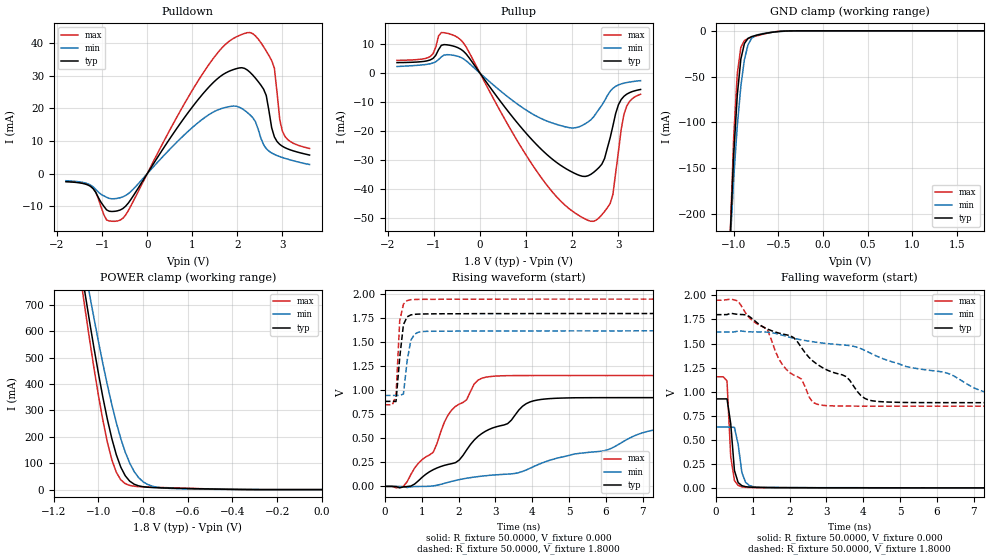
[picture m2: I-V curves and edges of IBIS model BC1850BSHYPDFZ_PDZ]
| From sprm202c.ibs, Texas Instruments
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|   Model BC1850BSHYPDFZ_PDZ
[Model]   BC1850BSHYPDFZ_PDZ
Model_type   I/O
Polarity   Non-Inverting
Enable   Active-Low
Vinl =   0.8500V
Vinh =   0.9800V
Vmeas =   0.9000V
Cref =  15.0000pF
Rref = 100.0000M
Vref =  0.000V
C_comp   1.3000pF   1.4700pF   0.9900pF
[Model Spec]
|   typ   min   max
Vinh   0.98V   0.86V   1.1V
Vinl   0.85V   0.70V   0.91V
[Temperature Range]   25.0000   0.1250k   -40.0000
[Voltage Range]   1.8000V   1.6200V   1.9500V
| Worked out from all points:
|   slope of the pulldown table from 0 to 0.27 V, typ, clamps not added: 46 ohm
|   slope of the pullup table from 0 to 0.27 V, typ, clamps not added: 44.9 ohm
|   GND clamp passes 1 mA (typ) near -0.52 V on its own axis
|   POWER clamp passes 1 mA (typ) near -0.40 V on its own axis
|   rising waveform, R_fixture 50.0000, V_fixture 0.000: 20-80 % time 2.15ns typ, 3.4ns min, 1.36ns max; typ from 0 V to 0.924 V
|   rising waveform, R_fixture 50.0000, V_fixture 1.8000: 20-80 % time 141ps typ, 150ps min, 87.9ps max; typ from 0.885 V to 1.8 V
|   falling waveform, R_fixture 50.0000, V_fixture 0.000: 20-80 % time 128ps typ, 165ps min, 115ps max; typ from 0.924 V to 0 V
|   falling waveform, R_fixture 50.0000, V_fixture 1.8000: 20-80 % time 2.09ns typ, 3.37ns min, 1.38ns max; typ from 1.8 V to 0.885 V
[Pulldown]
| voltage   I(typ)   I(min)   I(max)
-1.8V     -2.432mA   -2.13mA    -2.324mA
-1.2V     -4.535mA   -3.994mA   -4.328mA
-900mV    -11.04mA   -7.186mA   -14.12mA
-540mV    -10.64mA   -7.052mA   -13.61mA
1.32V     25.76mA    17.6mA     32.41mA
2.22V     31.69mA    18.71mA    43.1mA
2.58V     25.85mA    8.892mA    38.8mA
2.76V     14.03mA    6.343mA    34.57mA
2.82V     11.26mA    5.911mA    32.25mA
2.94V     8.959mA    5.236mA    16.41mA
3.06V     7.924mA    4.688mA    11.3mA
3.6V      5.706mA    2.822mA    7.711mA
[Pullup]
| voltage   I(typ)   I(min)   I(max)
-1.8V     3.669mA    2.32mA     4.446mA
-1.08V    4.598mA    3.276mA    5.779mA
-840mV    9.631mA    5.639mA    14.06mA
-420mV    8.322mA    5.5mA      11.54mA
1.32V     -26.18mA   -15.62mA   -35.92mA
1.98V     -34.04mA   -18.91mA   -47.41mA
2.4V      -34.97mA   -16.12mA   -51.17mA
2.64V     -31.45mA   -11.07mA   -48.94mA
2.82V     -22.35mA   -6.26mA    -45.06mA
2.88V     -18.23mA   -5.221mA   -41.92mA
3.12V     -7.968mA   -3.432mA   -14.2mA
3.48V     -5.616mA   -2.562mA   -7.289mA
[GND_clamp]
| voltage   I(typ)   I(min)   I(max)
-1.8V     -5.333A    -4.658A    -5.852A
-1.04V    -226.9mA   -235.1mA   -226.4mA
-1V       -135.8mA   -161.8mA   -116.3mA
-960mV    -70.57mA   -104.3mA   -47.27mA
-920mV    -30.97mA   -60.68mA   -18.06mA
-880mV    -13.88mA   -31.39mA   -10.61mA
-840mV    -8.324mA   -15.39mA   -8.431mA
-800mV    -6.322mA   -8.275mA   -7.135mA
-720mV    -4.296mA   -3.956mA   -4.93mA
-600mV    -2.054mA   -1.978mA   -2.087mA
-360mV    -85.5uA    -157.2uA   -38.41uA
1.8V      8.754nA    3.628uA    12.16nA
[POWER_clamp]
| voltage   I(typ)   I(min)   I(max)
-1.8V     5.299A     4.889A     5.644A
-1.08V    850.2mA    929.8mA    802mA
-1.06V    742mA      833.5mA    683.6mA
-1.04V    636.8mA    739.4mA    568.9mA
-1V       438.8mA    559.8mA    355.8mA
-960mV    265.5mA    395.4mA    178.9mA
-940mV    192.5mA    321mA      112.5mA
-920mV    131.7mA    253.1mA    65.29mA
-880mV    52.26mA    141.7mA    22.44mA
-820mV    14.13mA    45.17mA    11.23mA
-740mV    7.184mA    9.386mA    8.475mA
0V        8.78nA     22.3nA     13.47nA
[Ramp]
| variable   typ   min   max
dV/dt_r   0.5546/2.1311n   0.3780/3.4669n   0.6926/1.3432n
dV/dt_f   0.5489/2.0680n   0.4028/3.4327n   0.6605/1.3638n
R_load = 50.0000
[Rising Waveform]
R_fixture = 50.0000
V_fixture = 0.000
V_fixture_min = 0.000
V_fixture_max = 0.000
| time   V(typ)   V(min)   V(max)
0s        534nV      1.078uV    250.2nV
505.1ps   -4.683mV   -4.244mV   1.036mV
909.1ps   57.65mV    -787.7uV   240.4mV
1.313ns   173.6mV    4.868mV    355.3mV
1.616ns   218.9mV    31.42mV    668.8mV
1.919ns   247.3mV    61.89mV    833.2mV
2.626ns   548.7mV    106.5mV    1.125V
4.242ns   905.4mV    239.9mV    1.154V
7.374ns   924.2mV    591.4mV    1.154V
10ns      924.3mV    630.1mV    1.154V
[Rising Waveform]
R_fixture = 50.0000
V_fixture = 1.8000
V_fixture_min = 1.6200
V_fixture_max = 1.9500
| time   V(typ)   V(min)   V(max)
0s        885.2mV    946.9mV    849.1mV
202ps     885.5mV    946.9mV    849.3mV
303ps     884mV      947.4mV    942mV
404ps     1.34V      946.8mV    1.724V
505.1ps   1.685V     962.5mV    1.898V
606.1ps   1.766V     1.31V      1.935V
707.1ps   1.786V     1.523V     1.944V
808.1ps   1.792V     1.586V     1.946V
1.01ns    1.795V     1.612V     1.948V
10ns      1.8V       1.62V      1.95V
[Falling Waveform]
R_fixture = 50.0000
V_fixture = 0.000
V_fixture_min = 0.000
V_fixture_max = 0.000
| time   V(typ)   V(min)   V(max)
0s        924.3mV    631.6mV    1.154V
303ps     925mV      631.6mV    1.111V
404ps     667.9mV    631.6mV    324.7mV
505.1ps   180.1mV    628.1mV    76.94mV
606.1ps   54.79mV    451.5mV    25.63mV
707.1ps   22.43mV    159.9mV    10.34mV
808.1ps   12.2mV     57.3mV     5.119mV
909.1ps   8.3mV      24.57mV    3.619mV
1.212ns   4.003mV    6.421mV    1.853mV
10ns      3.8uV      139.5uV    249.9nV
[Falling Waveform]
R_fixture = 50.0000
V_fixture = 1.8000
V_fixture_min = 1.6200
V_fixture_max = 1.9500
| time   V(typ)   V(min)   V(max)
0s        1.8V       1.62V      1.95V
606.1ps   1.802V     1.629V     1.94V
1.414ns   1.648V     1.617V     1.631V
1.818ns   1.598V     1.585V     1.275V
2.323ns   1.458V     1.538V     1.131V
2.727ns   1.291V     1.513V     872.1mV
3.535ns   1.156V     1.482V     849.8mV
4.242ns   904.8mV    1.391V     849.1mV
7.475ns   885.2mV    982.8mV    849.1mV
10ns      885.2mV    948.6mV    849.1mV
